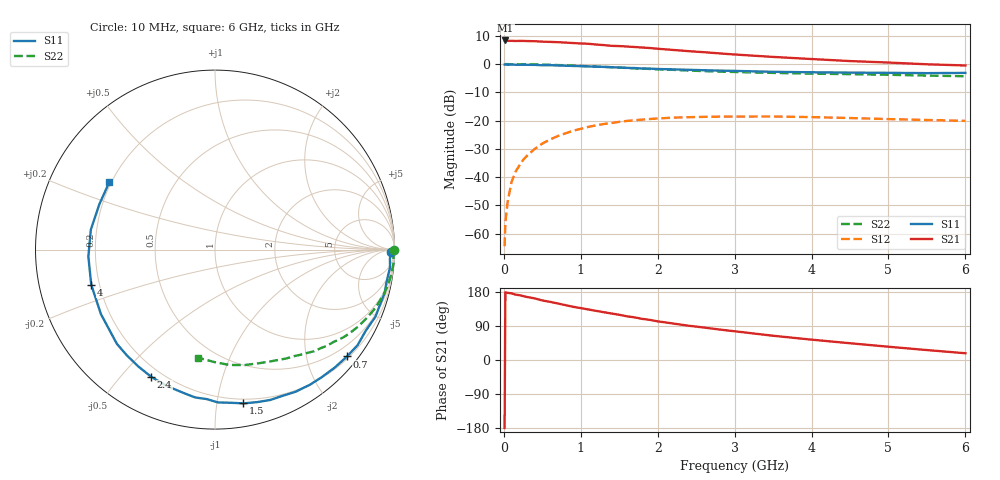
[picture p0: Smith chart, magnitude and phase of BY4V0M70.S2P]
! SIEMENS Small Signal Semiconductors
! BFY420
! Si NPN RF SIEGET Grounded Emitter Transistor in MICRO-X
! VCE = 4 V  IC = 0.7 mA
! Common Emitter S-Parameters:  October  1996
# GHz  S  MA  R  50
!  f  S11  S21  S12  S22
! GHz  MAG  ANG  MAG  ANG  MAG  ANG  MAG  ANG
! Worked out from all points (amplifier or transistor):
!   36 points, 10 MHz to 6 GHz, reference 50 ohm
!   highest |S21| = 8.4 dB at 20 MHz (marker M1)
!   |S21| within 3 dB of that: start of sweep to 2.031 GHz
!   unconditionally stable (mu >= 1): 4.629 GHz to end of sweep
!   at 250 MHz: K = 0.06, MSG = 21.1 dB, |S12| = -33.9 dB
!   at 1.4 GHz: K = 0.16, MSG = 13.7 dB, |S12| = -20.9 dB
!   at 6 GHz: K = 1.41, MAG = 6.0 dB, |S12| = -20.1 dB
!   S11 on the Smith chart (normalised r, x): 10 MHz: 71, -40; 700 MHz: 0.25, -2.80; 1.5 GHz: 0.17, -1.19; 2.4 GHz: 0.16, -0.61; 4 GHz: 0.17, -0.13; 6 GHz: 0.19, +0.28
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0.01  0.9789 -0.7  2.618 -179.3  0.0006 88.1  0.9999 -0.2
0.02  0.981 -1.4  2.62 178.7  0.0016 70.8  0.9999 -0.6
0.05  0.9757 -2.9  2.574 177.2  0.0037 88.1  0.9987 -1.2
0.1  0.9801 -5.9  2.58 175.9  0.0082 85.3  0.9952 -2.6
0.15  0.9749 -8.6  2.564 172.6  0.0123 82.8  0.9966 -3.8
0.25  0.9757 -14.2  2.572 168.7  0.0201 79.3  0.9944 -6.3
0.4  0.9687 -22.8  2.54 162.6  0.0314 76.3  0.9868 -10.1
0.5  0.9538 -28.3  2.495 157.1  0.0392 73.2  0.9798 -12.5
0.7  0.9462 -39.0  2.443 149.2  0.0532 66.6  0.9616 -17.3
0.9  0.9269 -49.9  2.357 140.4  0.0663 59.4  0.94 -21.9
1.1  0.9105 -60.4  2.288 133.3  0.0775 53.5  0.9158 -26.3
1.5  0.8713 -79.5  2.084 119.3  0.095 42.3  0.8678 -34.1
1.8  0.8343 -93.1  1.964 108.5  0.1041 35.2  0.8299 -39.2
2.2  0.8061 -109.3  1.78 96.3  0.1127 26.5  0.7912 -45.7
2.4  0.793 -116.6  1.696 90.5  0.115 23.0  0.7685 -48.7
2.8  0.767 -129.9  1.548 80.5  0.1176 16.4  0.7355 -54.1
3.5  0.7301 -150.6  1.34 64.0  0.1182 7.6  0.6982 -62.8
4  0.7167 -164.2  1.229 53.7  0.1153 3.2  0.6782 -69.1
4.5  0.7066 -176.9  1.131 44.2  0.1111 -0.4  0.6641 -75.6
5  0.7007 170.9  1.065 35.0  0.1065 -2.0  0.6476 -83.0
5.5  0.6921 158.7  0.992 26.2  0.1026 -2.6  0.6264 -90.4
6  0.6988 147.4  0.945 17.8  0.0989 -1.2  0.6097 -98.7
